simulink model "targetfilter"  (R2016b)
settings: Solver=ode45  StartTime=0.0  StopTime=5  RelTol=1e-3  EnableMultiTasking=on
PreLoadFcn:
  | L = 0.01;
  | eta = 0.1;
  | Kp = 21.791;
  | Ti = 0.02;
  | Td = 0.005;
  | Tf = 0.1;
  | Kf = 3;

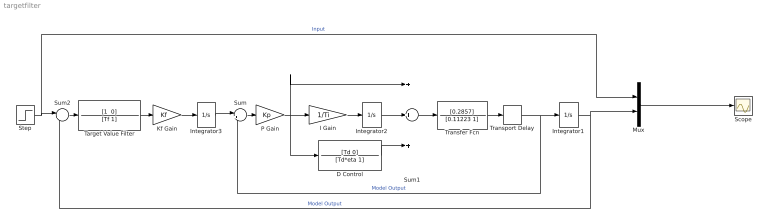
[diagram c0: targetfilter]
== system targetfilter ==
  D Control : TransferFcn  Numerator=[Td 0]  Denominator=[Td*eta 1]
  I Gain : Gain  Gain=1/Ti
  Integrator1 : Integrator
  Integrator2 : Integrator
  Integrator3 : Integrator
  Kf Gain : Gain  Gain=Kf
  Mux : Mux  Inputs=2
  P Gain : Gain  Gain=Kp
  Scope : Scope
  Step : Step  SampleTime=0.02
  Sum : Sum  Inputs=|+-
  Sum1 : Sum  Inputs=+++
  Sum2 : Sum  Inputs=|+-
  Target Value Filter : TransferFcn  Numerator="[1  0]"  Denominator=[Tf 1]
  Transfer Fcn : TransferFcn  Numerator=[0.2857]  Denominator=[0.11223 1]
  Transport Delay : TransportDelay  DelayTime=L
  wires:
  Transfer Fcn/1 -> Transport Delay/1
  Mux/1 -> Scope/1
  Transport Delay/1 -> Sum/2, Integrator1/1  "Model Output"
  Integrator2/1 -> Sum1/2
  D Control/1 -> Sum1/3
  Sum1/1 -> Transfer Fcn/1
  P Gain/1 -> Sum1/1, I Gain/1, D Control/1
  Sum/1 -> P Gain/1
  I Gain/1 -> Integrator2/1
  Step/1 -> Sum2/1, Mux/1  "Input"
  Sum2/1 -> Target Value Filter/1
  Integrator1/1 -> Mux/2, Sum2/2  "Model Output"
  Target Value Filter/1 -> Kf Gain/1
  Kf Gain/1 -> Integrator3/1
  Integrator3/1 -> Sum/1
